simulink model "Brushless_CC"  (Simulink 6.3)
settings: Solver=ode45  StartTime=0.0  StopTime=10.0  RelTol=1e-6  AbsTol=1e-6
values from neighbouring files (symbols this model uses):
  b = 0.8*Nm*s/rad    (= 0.8)    [Brushless_CC_CtrlOpt.m]
  Cr = 0*N*m    (= 0)    [Brushless_CC_CtrlOpt.m]
  Imax = 5.6*Amp    (= 5.6)    [Brushless_CC_CtrlOpt.m]
  J = 8*kg*m^2    (= 8)    [Brushless_CC_CtrlOpt.m]
  Ke = 10*N*m/Amp    (= 10)    [Brushless_CC_CtrlOpt.m]
  La = 0.1*Henry    (= 0.1)    [Brushless_CC_CtrlOpt.m]
  Ra = 8*Ohm    (= 8)    [Brushless_CC_CtrlOpt.m]

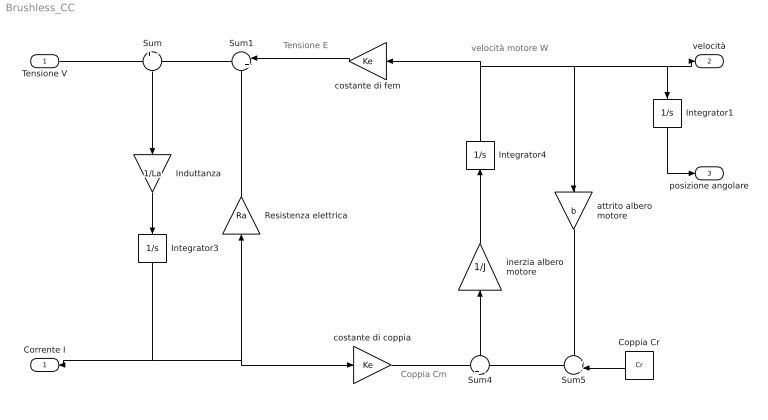
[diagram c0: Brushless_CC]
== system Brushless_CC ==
  note: Tensione E
  note: velocità motore W
  note: Coppia Cm
  Tensione V : Inport
  Coppia Cr : Constant  Orientation=left  Value=Cr
  Induttanza : Gain  Orientation=down  Gain=1/La
  Integrator1 : Integrator  Orientation=down
  Integrator3 : Integrator  Orientation=down  LimitOutput=on  UpperSaturationLimit=Imax  LowerSaturationLimit=-Imax
  Integrator4 : Integrator  Orientation=up
  Resistenza elettrica : Gain  Orientation=up  Gain=Ra
  Sum : Sum  Orientation=down  Inputs=+|-
  Sum1 : Sum  Orientation=left  Inputs=|++
  Sum4 : Sum  Orientation=up  Inputs=+|-
  Sum5 : Sum  Orientation=left  Inputs=++|
  attrito albero motore : Gain  Orientation=down  Gain=b
  costante di coppia : Gain  Gain=Ke
  costante di fem : Gain  Orientation=left  Gain=Ke
  inerzia albero motore : Gain  Orientation=up  Gain=1/J
  Corrente I : Outport  Orientation=left
  velocità : Outport  Port=2
  posizione angolare : Outport  Port=3
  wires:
  Sum/1 -> Induttanza/1
  Induttanza/1 -> Integrator3/1
  Resistenza elettrica/1 -> Sum1/2
  Sum4/1 -> inerzia albero motore/1
  inerzia albero motore/1 -> Integrator4/1
  Sum5/1 -> Sum4/2
  attrito albero motore/1 -> Sum5/1
  Integrator4/1 -> costante di fem/1, Integrator1/1, velocità/1, attrito albero motore/1
  costante di fem/1 -> Sum1/1
  Coppia Cr/1 -> Sum5/2
  Integrator3/1 -> Resistenza elettrica/1, costante di coppia/1, Corrente I/1
  Sum1/1 -> Sum/2
  costante di coppia/1 -> Sum4/1
  Tensione V/1 -> Sum/1
  Integrator1/1 -> posizione angolare/1
